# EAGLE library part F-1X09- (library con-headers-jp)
FEMALE HEADER
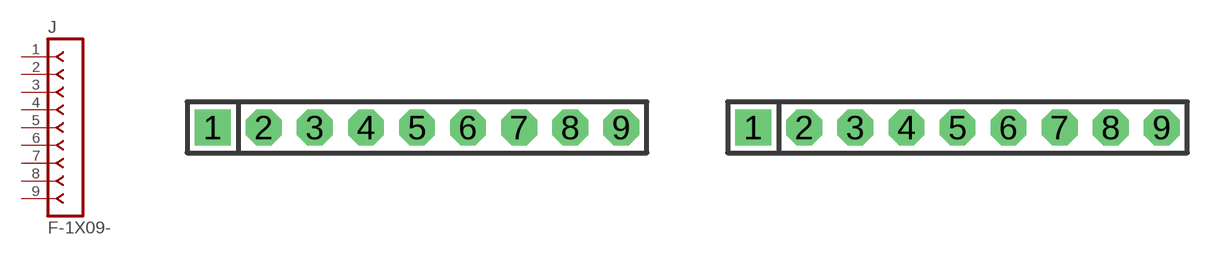
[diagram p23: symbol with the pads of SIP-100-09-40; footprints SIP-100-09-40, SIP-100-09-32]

Designator prefix J

## F-1X09-SIP-100-40  [SIP-100-09-40]
1  1  pas
2  2  pas
3  3  pas
4  4  pas
5  5  pas
6  6  pas
7  7  pas
8  8  pas
9  9  pas

## F-1X09-SIP-100-32  [SIP-100-09-32]
Pads as for SIP-100-09-40

## F-1X09-SIP-100-32Y  [SIP-100-09-32Y]
Pads as for SIP-100-09-40

## F-1X09-SIP-100-40Y  [SIP-100-09-40Y]
Pads as for SIP-100-09-40

## Footprint SIP-100-09-40 (pad centres in mm)
SIP Header - 0.1", 40 mil drill
drill 1.016 pad 1.778 square: 1 -10.16,0
drill 1.016 pad 1.778 octagon: 2 -7.62,0; 3 -5.08,0; 4 -2.54,0; 5 0,0; 6 2.54,0; 7 5.08,0; 8 7.62,0; 9 10.16,0

## Footprint SIP-100-09-32 (pad centres in mm)
SIP Header - 0.1", 32 mil drill
drill 0.813 pad 1.778 square: 1 -10.16,0
drill 0.813 pad 1.778 octagon: 2 -7.62,0; 3 -5.08,0; 4 -2.54,0; 5 0,0; 6 2.54,0; 7 5.08,0; 8 7.62,0; 9 10.16,0

## Footprint SIP-100-09-32Y (pad centres in mm)
SIP Header - 0.1", 32 mil drill
drill 0.813 long: 1 -10.16,0; 2 -7.62,0; 3 -5.08,0; 4 -2.54,0; 5 0,0; 6 2.54,0; 7 5.08,0; 8 7.62,0; 9 10.16,0

## Footprint SIP-100-09-40Y (pad centres in mm)
SIP Header - 0.1", 40 mil drill
drill 1.016 long: 1 -10.16,0; 2 -7.62,0; 3 -5.08,0; 4 -2.54,0; 5 0,0; 6 2.54,0; 7 5.08,0; 8 7.62,0; 9 10.16,0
